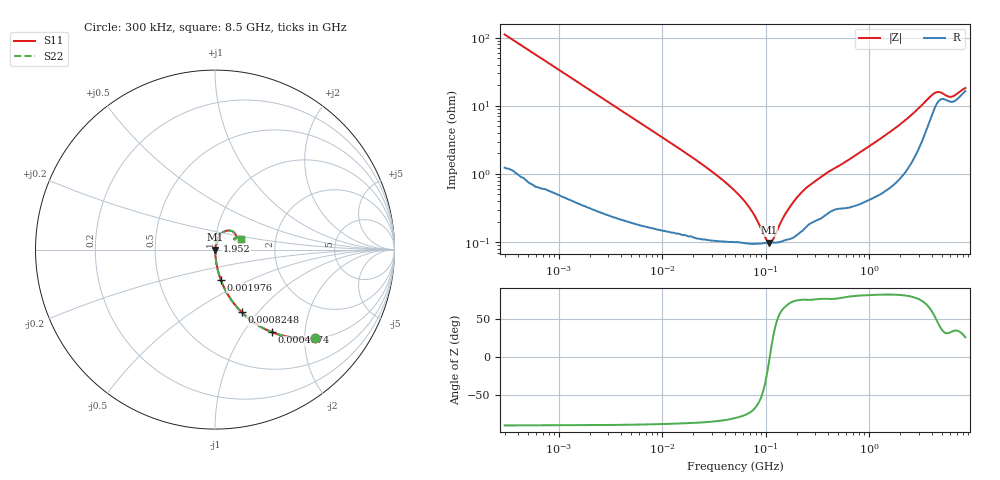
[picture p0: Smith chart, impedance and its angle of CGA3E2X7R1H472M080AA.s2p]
! S-parameter Generated by TDK Corporation
! Copyright(C) 2015 TDK Corporation.
! All Rights Reserved.
! TDK P/N: CGA3E2X7R1H472M080AA (Multilayer Ceramic Chip Capacitors)
! Property: C=4.7nF
! Size(LxWxT): 1.6x0.8x0.8mm, 0.063x0.031x0.031inches
! Model Type: s2p (Touchstone File Format Version 1.0)
! Frequency: DC=Yes Start=0.3MHz Stop=8500MHz 225points Log-sweep
! Note:
! Model Generated on Jun. 23, 2015
! Hash(MD5):
! Port Assignments:
!  1 ---| |--- 2
! Applicable Conditions:
!  Temperature = 25 degC
!  DC Bias Voltage = 0 V
!  Small Signal Operation
! Terms and conditions regarding TDK Simulation Models
! (1)This simulation model is being provided solely for informational purposes. Please refer to the specifications of the products in terms of detailed characteristics of such products.
! (2)In no event shall TDK Corporation of any of its subsidiaries be liable for any loss or damage arising, directly or indirectly,
!  From any information contained in this simulation model, including, but not limited to loss or damages arising from any inaccuracies, omissions or errors in connection with such information.
! (3)Any and all copyrights on this simulation model are owned by TDK Corporation.
!  Duplication or redistribution of this simulation model without prior written permission from TDK Corporation is prohibited.
! (4)This simulation model is subject to any modification or change without any prior notice.
! (5)Neither TDK Corporation nor any of its subsidiaries shall make any warranty, express or implied,
!  Including but not limited to the correctness, implied warranties of merchantability and fitness for a particular purpose with respect to this simulation models.
! (6)The use of this simulation model shall be deemed to have consented to the terms and conditions hereof.
# MHz S MA R 50
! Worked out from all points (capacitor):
!   224 points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, 300 kHz to 8.5 GHz, reference 50 ohm
!   read as one part in series: C = 4.72 nF near 314.1 kHz
!   lowest |Z| = 98.3 mohm at 107.8 MHz (marker M1)
!   series resonance near 109.5 MHz, so ESL is about 450 pH
!   S11 on the Smith chart (normalised r, x): 300 kHz: 1.02, -2.24; 497.4 kHz: 1.02, -1.36; 824.8 kHz: 1.01, -0.82; 1.976 MHz: 1.01, -0.35; 1.952 GHz: 1.02, +0.10; 8.5 GHz: 1.33, +0.16
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0.3  0.7419 -41.5  0.6623 47.9  0.6623 47.9  0.7419 -41.5
0.4974407  0.5592 -55.3  0.8227 34.0  0.8227 34.0  0.5592 -55.3
0.8248242  0.3787 -67.0  0.9204 22.3  0.9204 22.3  0.3787 -67.0
1.72111  0.1939 -77.8  0.9777 11.2  0.9777 11.2  0.1939 -77.8
1.975628  0.17 -79.2  0.9824 9.8  0.9824 9.8  0.17 -79.2
9.430415  0.03655 -85.6  0.9978 2.1  0.9978 2.1  0.03655 -85.6
29.76236  0.01104 -83.9  0.9989 0.6  0.9989 0.6  0.01104 -83.9
51.67171  0.005438 -79.2  0.999 0.3  0.999 0.3  0.005438 -79.2
71.28712  0.003047 -71.8  0.9991 0.2  0.9991 0.2  0.003047 -71.8
98.34885  0.001187 -35.6  0.999 0.0  0.999 0.0  0.001187 -35.6
107.8202  0.0009817 -5.7  0.999 0.0  0.999 0.0  0.0009817 -5.7
118.2037  0.001102 26.9  0.999 -0.0  0.999 -0.0  0.001102 26.9
148.7505  0.002335 63.4  0.999 -0.1  0.999 -0.1  0.002335 63.4
187.1913  0.003966 72.6  0.9988 -0.2  0.9988 -0.2  0.003966 72.6
283.1228  0.007311 74.2  0.998 -0.4  0.998 -0.4  0.007311 74.2
1551.304  0.04015 79.1  0.9932 -2.3  0.9932 -2.3  0.04015 79.1
1952.199  0.05193 77.9  0.9905 -2.9  0.9905 -2.9  0.05193 77.9
3091.568  0.09363 69.4  0.971 -5.2  0.971 -5.2  0.09363 69.4
4265.177  0.1401 47.3  0.9107 -6.5  0.9107 -6.5  0.1401 47.3
4675.929  0.1429 37.3  0.8906 -5.6  0.8906 -5.6  0.1429 37.3
6161.135  0.1215 28.7  0.8952 -3.7  0.8952 -3.7  0.1215 28.7
8500  0.157 21.7  0.8561 -3.9  0.8561 -3.9  0.157 21.7
